FUNCTION_BLOCK FB_Simulation

VAR
	fbVisu						: FB_Visu;	

	// =============== 特定位置参数 ======================
	SimuParam					: SimuParameter;
	
	// =============== 四个物料代表灰色和绿色随机切换的标志位 ======================
	ArrColorSwitch				: ARRAY[1..4] OF BOOL;

	// =============== 气缸位置状态 ======================
	bClampAtBase		AT %Q*	: BOOL;						// 如果为TRUE，则正位气缸在基始位置
	bClampAtWork		AT %Q*	: BOOL;						// 如果为TRUE，则正位气缸在目标位置
	bBarrierAtBase		AT %Q*	: BOOL;						// 如果为TRUE，则栏杆气缸在基始位置
	bBarrierAtWork		AT %Q*	: BOOL;						// 如果为TRUE，则栏杆气缸在目标位置
	bMetalAtBase		AT %Q*	: BOOL;						// 如果为TRUE，则金属分拣气缸在基始位置
	bMetalAtWork		AT %Q*	: BOOL;						// 如果为TRUE，则金属分拣气缸在目标位置
	bPlasticAtBase		AT %Q*	: BOOL;						// 如果为TRUE，则塑料分拣气缸在基始位置
	bPlasticAtWork		AT %Q*	: BOOL;						// 如果为TRUE，则塑料分拣气缸在目标位置
	
	// =============== 气缸温度数据 =========================
	bReset				AT %I*	: BOOL;						// 如果为TRUE，则复位气缸温度
	fClampTempCurrent	AT %Q*	: LREAL;					// 正位气缸的实际温度
	fClampTempMax		AT %Q*	: LREAL;					// 正位气缸的设定最大温度
	fClampTempMin		AT %Q*	: LREAL;					// 正位气缸的设定最小温度
	fBarrierTemp		AT %Q*	: LREAL;					// 栏杆气缸的温度

	// =============== 检测物料的传感器信号 ==============
	bBarrierSensor		AT %Q*	: BOOL;						// 如果为TRUE，则栏杆前检测到物料
	bMetalSensor		AT %Q*	: BOOL;						// 如果为TRUE，则检测到金属物料
	bPlasticSensor		AT %Q*	: BOOL;						// 如果为TRUE，则检测到塑料物料

	// =============== 特定点坐标以及物料坐标 ===================
	fYClamp						: LREAL;					// 正位气缸的纵坐标
	fYBarrier					: LREAL;					// 栏杆气缸的纵坐标
	fYMetal						: LREAL;					// 金属分拣气缸的纵坐标
	fYPlastic					: LREAL;					// 塑料分拣气缸的纵坐标
	fBoxX						: ARRAY[1..4] OF LREAL;		// 物料的X轴坐标
	fBoxY						: ARRAY[1..4] OF LREAL;		// 物料的Y轴坐标
	
	bTempUp						: BOOL;						// 如果为TRUE，则升高正位气缸的温度
	fbTimerTempChange			: TON;						// 升高温度过程所需要的 TON 功能块
	tTempChange					: TIME 	:= T#1S;			// 升高温度过程时间
END_VAR



// 气缸位置检测
CylinderSensorSignal();

// 物料位置检测
SelectLightSensorSignal();

//温度处理
Temperatures();

// HMI
General_Visu();

METHOD PRIVATE CylinderSensorSignal
VAR_INPUT
END_VAR
// =========================================================
// 根据 SimuParam 中的参数判断各个气缸在基始位置或者目标位置
	
	bClampAtWork 	:= (fYClamp = SimuParam.cClampAtWork);
	bClampAtBase 	:= (fYClamp = SimuParam.cClampAtBase);
	bBarrierAtWork 	:= (fYBarrier = SimuParam.cBarrierAtWork);
	bBarrierAtBase 	:= (fYBarrier = SimuParam.cBarrierAtBase);
	bMetalAtWork 	:= (fYMetal < SimuParam.cMetalAtWorkMin) AND (fYMetal > SimuParam.cMetalAtWorkMax);
	bMetalAtBase 	:= (fYMetal = SimuParam.cMetalAtBase);
	bPlasticAtWork 	:= (fYPlastic < SimuParam.cPlasticAtWorkMin) AND (fYPlastic > SimuParam.cPlasticAtWorkMax);
	bPlasticAtBase 	:= (fYPlastic = SimuParam.cPlasticAtBase);

// =========================================================
END_METHOD

METHOD PRIVATE General_Visu
VAR_INPUT
END_VAR

VAR

END_VAR
// =========================================================
// 从 fbVisu 的属性当中传递数据到功能块当中
fYClamp			:= fbVisu.P_fYClamp;
fYBarrier		:= fbVisu.P_fYBarrier;
fYMetal			:= fbVisu.P_fYMetal;
fYPlastic		:= fbVisu.P_fYPlastic;
fBoxX			:= fbVisu.P_ArrfBoxX;
fBoxY			:= fbVisu.P_ArrfBoxY;
ArrColorSwitch	:= fbVisu.P_ArrChangeColor;

fbVisu();

// =========================================================
END_METHOD

METHOD PRIVATE SelectLightSensorSignal
VAR_INPUT
END_VAR

VAR
	
END_VAR
// =========================================================
// 检测每个物料是否被栏杆前的传感器检测到/被金属传感器检测到/被塑料传感器检测到
	
	bBarrierSensor := 	( (fBoxY[1] >= SimuParam.cSensorsBoxesY) AND (fBoxX[1] > SimuParam.cBarrierSensorBox1Xmin) 	AND (fBoxX[1] < SimuParam.cBarrierSensorBox1Xmax) )
					OR 	( (fBoxY[2] >= SimuParam.cSensorsBoxesY) AND (fBoxX[2] > SimuParam.cBarrierSensorBox2Xmin) 	AND (fBoxX[2] < SimuParam.cBarrierSensorBox2Xmax) )
					OR 	( (fBoxY[3] >= SimuParam.cSensorsBoxesY) AND (fBoxX[3] > SimuParam.cBarrierSensorBox3Xmin) 	AND (fBoxX[3] < SimuParam.cBarrierSensorBox3Xmax) )
					OR 	( (fBoxY[4] >= SimuParam.cSensorsBoxesY) AND (fBoxX[4] > SimuParam.cBarrierSensorBox4Xmin) 	AND (fBoxX[4] < SimuParam.cBarrierSensorBox4Xmax) );
	

	bMetalSensor := 	( (fBoxY[1] >= SimuParam.cSensorsBoxesY) AND (fBoxX[1] > SimuParam.cMetalSensorBox1Xmin) 	AND (fBoxX[1] < SimuParam.cMetalSensorBox1Xmax)  AND (ArrColorSwitch[1] = TRUE))
					OR 	( (fBoxY[2] >= SimuParam.cSensorsBoxesY) AND (fBoxX[2] > SimuParam.cMetalSensorBox2Xmin) 	AND (fBoxX[2] < SimuParam.cMetalSensorBox2Xmax)  AND (ArrColorSwitch[2] = TRUE)) 
					OR 	( (fBoxY[3] >= SimuParam.cSensorsBoxesY) AND (fBoxX[3] > SimuParam.cMetalSensorBox3Xmin) 	AND (fBoxX[3] < SimuParam.cMetalSensorBox3Xmax)  AND (ArrColorSwitch[3] = TRUE))
					OR 	( (fBoxY[4] >= SimuParam.cSensorsBoxesY) AND (fBoxX[4] > SimuParam.cMetalSensorBox4Xmin) 	AND (fBoxX[4] < SimuParam.cMetalSensorBox4Xmax)  AND (ArrColorSwitch[4] = TRUE))  ;
					
	bPlasticSensor := 	( (fBoxY[1] >= SimuParam.cSensorsBoxesY) AND (fBoxX[1] > SimuParam.cPlasticSensorBox1Xmin) 	AND (fBoxX[1] < SimuParam.cPlasticSensorBox1Xmax) AND (ArrColorSwitch[1] = FALSE))
					OR 	( (fBoxY[2] >= SimuParam.cSensorsBoxesY) AND (fBoxX[2] > SimuParam.cPlasticSensorBox2Xmin) 	AND (fBoxX[2] < SimuParam.cPlasticSensorBox2Xmax) AND (ArrColorSwitch[2] = FALSE))
					OR 	( (fBoxY[3] >= SimuParam.cSensorsBoxesY) AND (fBoxX[3] > SimuParam.cPlasticSensorBox3Xmin) 	AND (fBoxX[3] < SimuParam.cPlasticSensorBox3Xmax) AND (ArrColorSwitch[3] = FALSE))
					OR 	( (fBoxY[4] >= SimuParam.cSensorsBoxesY) AND (fBoxX[4] > SimuParam.cPlasticSensorBox4Xmin) 	AND (fBoxX[4] < SimuParam.cPlasticSensorBox4Xmax) AND (ArrColorSwitch[4] = FALSE));

// =========================================================
END_METHOD

METHOD PRIVATE Temperatures
VAR_INPUT
END_VAR
// =========================================================

// 复位温度
IF bReset THEN
	fClampTempCurrent 	:= 0;
	fBarrierTemp 		:= 0;
END_IF

// 从 SimuParam 中传递温度参数数据

	fClampTempMax 		:= SimuParam.cClampTempMax;
	fClampTempMin 		:= SimuParam.cClampTempMin;
	fClampTempCurrent 	:= SimuParam.cClampTempCurrent;

// =========================================================
// 温度处理

	fbTimerTempChange(PT := tTempChange);
	
	IF NOT fbTimerTempChange.Q THEN
		fbTimerTempChange(IN := TRUE);
	END_IF
	
	IF fBarrierTemp >= SimuParam.cBarrierTempMax THEN
		bTempUp := FALSE;
	ELSIF fBarrierTemp <= SimuParam.cBarrierTempMin THEN
		bTempUp := TRUE;
	END_IF
	
	IF fbTimerTempChange.Q THEN
		
		fbTimerTempChange(IN := FALSE);
		
		IF bTempUp THEN
			fBarrierTemp := fBarrierTemp + SimuParam.cBarrierTempChange;
		ELSE
			fBarrierTemp := fBarrierTemp - SimuParam.cBarrierTempChange;
		END_IF
	END_IF

// =========================================================
END_METHOD

END_FUNCTION_BLOCK
